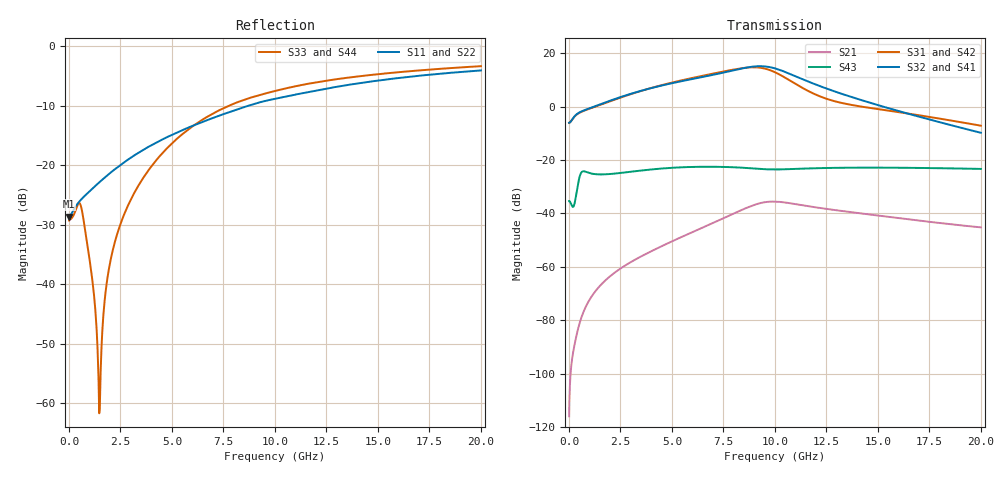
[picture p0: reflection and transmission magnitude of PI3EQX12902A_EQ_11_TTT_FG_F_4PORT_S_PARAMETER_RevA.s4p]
! NPort=4 DATA=2000 NOISE=0 GROUPDELAY=0 COMPLEX_DATAFORMAT=POLAR
! NumOfBlock=1 NumOfParam=0
! .MODEL Smodel S TSTONEFILE=PI3EQX12902A_EQ_11_TTT_FG_F_4PORT_S_PARAMETER_RevA.s4p TYPE=S
!  -- The above .MODEL line can be used for the S element in the netlist.
! The s parameter is extracted from the linear redriver, it is not bi-directional; only s(4,1)s(4,2) and s(3,1)s(3,2)
! should be the insertion loss
!Port definition:
!Port1 = input+
!Port2 = input-
!Port3 = output+
!Port4 = output-
# Hz S MA R  50
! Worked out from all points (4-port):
!   2000 points, 10 MHz to 20 GHz, reference 50 ohm
!   strongest paths, dB at 10 MHz, 5.01 GHz, 10.01 GHz, 15.01 GHz, 20 GHz:
!     S32: -6.0, 8.8, 14.3, 0.6, -9.8
!     S41: -6.0, 8.8, 14.2, 0.5, -9.8
!     S31: -6.0, 9.0, 12.9, -0.9, -7.1
!     S42: -6.0, 8.9, 12.7, -1.1, -7.2
!     S43: -35.3, -22.9, -23.5, -22.8, -23.3
!     S21: -116.0, -50.4, -35.6, -40.8, -45.2
!   lowest |S11| = -28.6 dB at 10 MHz (marker M1), VSWR 1.08, Z = 46.4 - j0.0607 ohm
!   |S11| at or under -10 dB: start of sweep to 8.715 GHz
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1e7  0.03704 -179.0  1.589e-06 51.9  0 0.0  0 0.0
     1.589e-06 51.9  0.03704 -179.0  0 0.0  0 0.0
     0.4991 1.2  0.4991 -178.8  0.03429 6.0  0.01709 -177.1
     0.4991 -178.8  0.4991 1.2  0.01709 -177.1  0.03429 6.0
5.78e9  0.2063 -111.9  0.004113 101.7  1.361e-06 -17.7  8.71e-07 89.3
        0.004113 101.8  0.2063 -111.9  8.738e-07 89.5  1.356e-06 -17.5
        3.309 -50.9  3.175 111.4  0.1986 -44.1  0.07365 147.1
        3.163 111.4  3.271 -51.5  0.07403 147.3  0.1981 -44.1
7.98e9  0.2871 -111.6  0.009884 76.9  7.174e-06 -81.7  4.367e-06 42.3
        0.009884 76.9  0.2871 -111.6  4.393e-06 42.3  7.149e-06 -81.4
        4.942 -110.4  4.774 51.5  0.3272 -65.8  0.07291 123.9
        4.748 51.4  4.869 -110.8  0.07339 123.8  0.3265 -65.8
9.26e9  0.3374 -113.6  0.01554 44.8  1.354e-05 -130.3  1.076e-05 -2.8
        0.01553 44.8  0.3374 -113.6  1.08e-05 -3.0  1.349e-05 -129.8
        5.381 -162.7  5.732 -0.1  0.3888 -76.3  0.0679 113.8
        5.685 -0.2  5.298 -163.1  0.06829 113.6  0.3884 -76.2
1.041e10  0.3738 -115.8  0.01625 8.5  1.521e-05 -169.7  1.614e-05 -55.5
          0.01621 8.5  0.3737 -115.8  1.614e-05 -55.7  1.518e-05 -169.1
          3.649 148.3  4.607 -52.6  0.4371 -83.8  0.0668 109.4
          4.558 -52.4  3.585 147.9  0.06709 109.1  0.437 -83.7
1.241e10  0.4366 -118.6  0.01235 -26.7  1.845e-05 161.2  1.878e-05 -121.3
          0.01233 -26.6  0.4366 -118.6  1.871e-05 -121.4  1.853e-05 161.8
          1.448 115.8  2.253 -109.6  0.51 -94.7  0.07092 96.8
          2.23 -109.2  1.41 115.6  0.07095 96.4  0.5103 -94.7
2e10  0.6254 -131.7  0.005466 -77.1  3.922e-05 51.1  1.784e-05 94.8
      0.005496 -77.0  0.6254 -131.7  1.772e-05 95.3  3.953e-05 51.2
      0.4405 35.0  0.3243 128.2  0.6793 -119.6  0.06841 46.2
      0.3254 129.0  0.4346 35.8  0.06831 46.1  0.6797 -119.6
